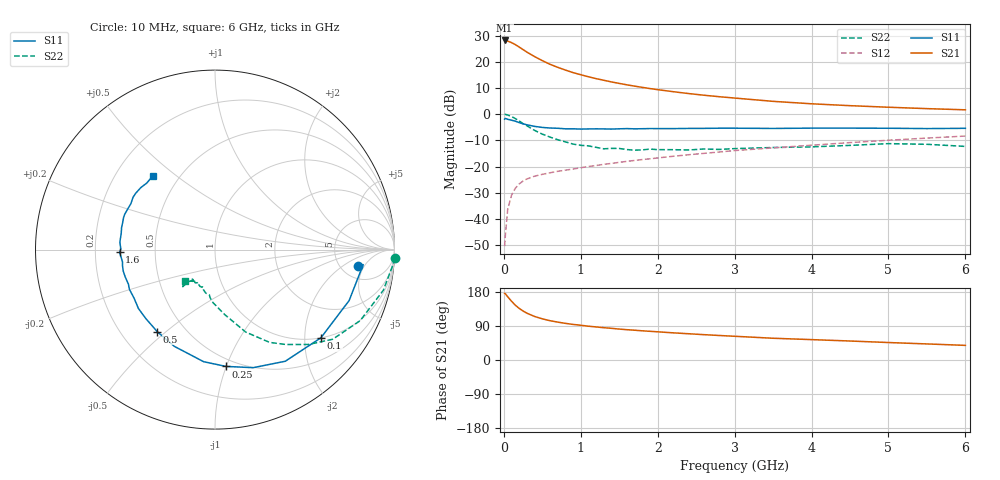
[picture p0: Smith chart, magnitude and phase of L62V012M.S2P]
!  INFINEON TECHNOLOGIES Small Signal Semiconductors
! BFR380L3 , Si-NPN RF-Transistor in TSLP-3-1
!  Vce=2 V,  Ic=12.5 mA
! Common Emitter S-Parameters:  07. March 2005
#  GHz  S  MA  R  50
! f  S11  S21  S12  S22
! GHz  Mag  Ang  Mag  Ang  Mag  Ang  Mag  Ang
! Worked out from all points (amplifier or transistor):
!   36 points, 10 MHz to 6 GHz, reference 50 ohm
!   highest |S21| = 28.2 dB at 10 MHz (marker M1)
!   |S21| within 3 dB of that: start of sweep to 224.2 MHz
!   unconditionally stable (mu >= 1): 2.022 GHz to 4.818 GHz
!   at 250 MHz: K = 0.29, MSG = 25.1 dB, |S12| = -25.5 dB
!   at 1.4 GHz: K = 0.91, MSG = 15.6 dB, |S12| = -18.8 dB
!   at 6 GHz: K = 0.97, MSG = 5.0 dB, |S12| = -8.4 dB
!   S11 on the Smith chart (normalised r, x): 10 MHz: 7.19, -3.74; 100 MHz: 1.00, -2.40; 250 MHz: 0.44, -1.00; 500 MHz: 0.35, -0.47; 1.6 GHz: 0.31, -0.01; 6 GHz: 0.36, +0.41
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0.01  0.8033 -6.6  25.69 175.6  0.003 84.4  1.003 -2.7
0.02  0.8299 -5.8  25.49 174.9  0.0049 87.4  0.9914 -5.7
0.05  0.7994 -20.8  25.03 166.9  0.0151 81.2  0.9648 -13.6
0.1  0.7679 -39.8  23.35 155.1  0.0283 72.4  0.9005 -26.1
0.15  0.735 -57.8  21.37 144.5  0.0385 64.0  0.8242 -37.3
0.2  0.6914 -72.1  19.18 136.1  0.0465 59.1  0.7422 -45.4
0.25  0.6535 -84.7  17.2 129.3  0.0528 54.6  0.6602 -53.2
0.3  0.6277 -95.8  15.38 123.5  0.0578 52.5  0.6002 -59.5
0.4  0.5847 -112.8  12.62 114.8  0.0654 48.7  0.4901 -69.6
0.5  0.5589 -125.2  10.57 108.7  0.0708 48.0  0.4161 -75.6
0.6  0.5442 -135.1  9.003 103.7  0.0758 47.5  0.3655 -81.6
0.7  0.5383 -142.4  7.879 100.0  0.0809 48.5  0.3251 -86.9
0.9  0.5258 -155.1  6.242 93.9  0.0895 50.1  0.2686 -95.9
1.1  0.5227 -163.0  5.195 89.2  0.1 52.2  0.2479 -101.9
1.4  0.5199 -172.5  4.135 83.6  0.1146 54.4  0.222 -109.0
1.6  0.531 -178.4  3.644 80.0  0.1255 55.7  0.2106 -116.9
2.2  0.5303 170.2  2.697 71.7  0.1569 58.6  0.2099 -121.8
2.8  0.54 160.5  2.16 64.7  0.1893 60.3  0.2121 -129.1
3.5  0.534 151.4  1.761 57.4  0.227 59.8  0.2309 -129.8
4.5  0.5419 144.5  1.456 50.1  0.2864 59.9  0.2534 -130.6
5.5  0.5311 135.7  1.278 42.4  0.3494 57.3  0.2659 -131.5
6  0.537 130.3  1.213 38.6  0.3821 55.6  0.2421 -133.7
